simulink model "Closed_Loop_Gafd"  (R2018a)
settings: Solver=ode23s  StartTime=0.0  StopTime=50  RelTol=1e-3  EnableMultiTasking=on
InitFcn:
  | init
StopFcn:
  | pl
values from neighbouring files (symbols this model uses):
  Cyb = -0.0245    [init.m]    (also in lqr_des.m)
  Cydel = [-0.24668,0.24668, 0.47413,-0.47413,0]/100    [init.m]    (also in lqr_des.m = [-0.24668,0.24668, 0.47413,-0.47413]/100)
  Cza = -0.073    [init.m]
  Czdel = [0.51664,0.51664,0.60478,0.60478,0.06]/100    [init.m]
  d2r = pi/180    (= 0.0174532925199)    [init.m]
  Mass = 198.32    [init.m]    (also in lqr_des.m)
  Qbar = 150    [init.m]    (also in lqr_des.m)
  r2d = 180/pi    (= 57.2957795131)    [init.m]    (also in pl.m)
  Sref = 79.069    [init.m]    (also in lqr_des.m)
  V0 = 822.8    [init.m]
undefined symbols (not defined in the file or in its folder): Abfp, Afla, Ardr, Avf, Bbfp, Bfla, Brdr, Bvf, Cbfp, Cfla, Crdr, Cvf, Dbfp, Dfla, Drdr, Dvf, K4axmix, Kpr, Kq

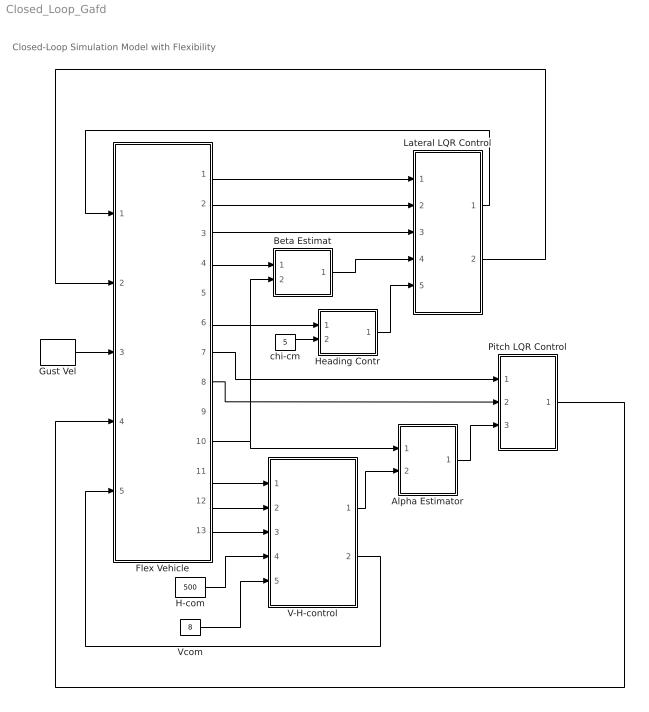
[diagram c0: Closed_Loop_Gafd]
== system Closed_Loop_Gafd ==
  note: Closed-Loop Simulation Model with Flexibility
  Alpha Estimator : Subsystem
  Beta Estimat : Subsystem
  Flex Vehicle : Subsystem
  Gust Vel : DiscretePulseGenerator  PulseType=Time based  Amplitude=160  Period=200  PulseWidth=0.05  PhaseDelay=8
  H-com : Constant  Value=500
  Heading Contr : Subsystem
  Lateral LQR Control : Subsystem
  Pitch LQR Control : Subsystem
  V-H-control : Subsystem
  Vcom : Constant  Value=8
  chi-cm : Constant  Value=5
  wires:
  chi-cm/1 -> Heading Contr/2(chi-cmd)
  Flex Vehicle/2(p) -> Lateral LQR Control/2(p)
  Flex Vehicle/3(r) -> Lateral LQR Control/3(r)
  Flex Vehicle/1(phi) -> Lateral LQR Control/1(phi)
  Flex Vehicle/4(Ny) -> Beta Estimat/1(Ydd)
  Flex Vehicle/6("chi ") -> Heading Contr/1(chi)
  Flex Vehicle/12(Nz) -> V-H-control/2(Az)
  Flex Vehicle/13(dH) -> V-H-control/3(dH)
  Flex Vehicle/11(V-dot) -> V-H-control/1(Vdot)
  Flex Vehicle/10(delt) -> Beta Estimat/2(delta), Alpha Estimator/1(delta)
  Alpha Estimator/1(alphat) -> Pitch LQR Control/3(alfa)
  V-H-control/1(Zdd-com) -> Alpha Estimator/2(Zdd)
  Pitch LQR Control/1(dQ) -> Flex Vehicle/4(dQ)
  Beta Estimat/1(bethat) -> Lateral LQR Control/4(bet)
  Lateral LQR Control/2(dR) -> Flex Vehicle/2(dR)
  Lateral LQR Control/1(dP) -> Flex Vehicle/1(dP)
  V-H-control/2(Throtle) -> Flex Vehicle/5(Ax-cmd)
  Flex Vehicle/8(q) -> Pitch LQR Control/2(q)
  Flex Vehicle/7(thet) -> Pitch LQR Control/1(thet)
  Heading Contr/1(phi-cmd) -> Lateral LQR Control/5(ph-cmd)
  H-com/1 -> V-H-control/4(H-comd)
  Vcom/1 -> V-H-control/5(Vcomd)
  Gust Vel/1 -> Flex Vehicle/3(Gust)

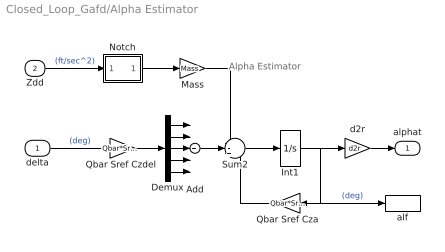
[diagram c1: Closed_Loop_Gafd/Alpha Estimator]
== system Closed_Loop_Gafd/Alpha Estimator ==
  note: Alpha Estimator
  delta : Inport
  Zdd : Inport  Port=2
  Add : Sum  Inputs=+++++
  Demux : Demux  Outputs=5
  Int1 : Integrator
  Mass : Gain  Gain=Mass
  Notch : Subsystem
  Qbar Sref Cza : Gain  Gain=Qbar*Sref*Cza
  "Qbar Sref Czdel " : Gain  Gain=Qbar*Sref*Czdel
  Sum2 : Sum  Inputs=--+
  alf : ToWorkspace  VariableName=alphat  SampleTime=-1
  d2r : Gain  Gain=d2r
  alphat : Outport
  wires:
  Demux/5 -> Add/5
  Demux/4 -> Add/4
  Demux/3 -> Add/3
  Demux/2 -> Add/2
  Demux/1 -> Add/1
  "Qbar Sref Czdel "/1 -> Demux/1
  delta/1 -> "Qbar Sref Czdel "/1  "(deg)"
  Sum2/1 -> Int1/1
  Int1/1 -> d2r/1, alf/1, Qbar Sref Cza/1  "(deg)"
  Qbar Sref Cza/1 -> Sum2/3
  Mass/1 -> Sum2/1
  d2r/1 -> alphat/1
  Add/1 -> Sum2/2
  Zdd/1 -> Notch/1(in)  "(ft/sec^2)"
  Notch/1(ou) -> Mass/1

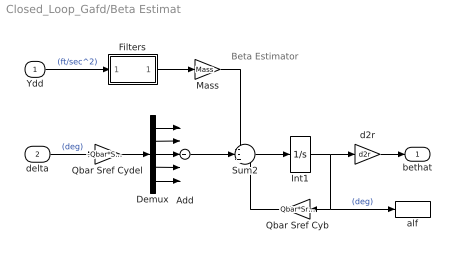
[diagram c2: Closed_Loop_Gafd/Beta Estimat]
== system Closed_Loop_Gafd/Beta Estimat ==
  note: Beta Estimator
  Ydd : Inport
  delta : Inport  Port=2
  Add : Sum  Inputs=+++++
  Demux : Demux  Outputs=5
  Filters : Subsystem
  Int1 : Integrator
  Mass : Gain  Gain=Mass
  Qbar Sref Cyb : Gain  Gain=Qbar*Sref*Cyb
  Qbar Sref Cydel : Gain  Gain=-Qbar*Sref*Cydel
  Sum2 : Sum  Inputs=--+
  alf : ToWorkspace  VariableName=bethat  SampleTime=-1
  d2r : Gain  Gain=d2r
  bethat : Outport
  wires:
  Add/1 -> Sum2/2
  d2r/1 -> bethat/1
  Mass/1 -> Sum2/1
  Ydd/1 -> Filters/1(In)  "(ft/sec^2)"
  Qbar Sref Cyb/1 -> Sum2/3
  Int1/1 -> d2r/1, alf/1, Qbar Sref Cyb/1  "(deg)"
  Sum2/1 -> Int1/1
  delta/1 -> Qbar Sref Cydel/1  "(deg)"
  Qbar Sref Cydel/1 -> Demux/1
  Demux/1 -> Add/1
  Demux/2 -> Add/2
  Demux/3 -> Add/3
  Demux/4 -> Add/4
  Demux/5 -> Add/5
  Filters/1(Ou) -> Mass/1

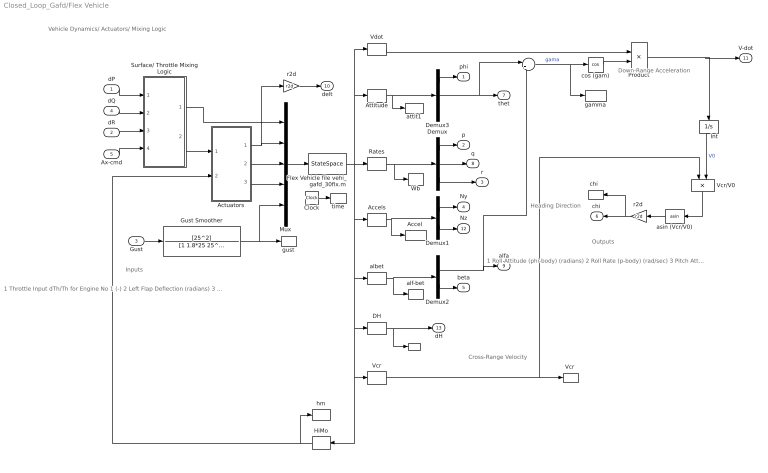
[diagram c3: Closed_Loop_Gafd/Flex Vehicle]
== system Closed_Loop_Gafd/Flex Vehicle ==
  note: 1 Roll Attitude (phi-body) (radians) 2 Roll Rate (p-body) (rad/sec) 3 Pitch Attitude (thet-bdy) (radians) 4 Pitch Rate (q-body) (rad/sec) 5 Yaw Attitude (psi-body) (radians) 6 Yaw Rate (r-body) (rad/sec) 7 Angle of attack, alfa, (radians) 8 Angle of sideslip, beta, (radian) 9 Change in Altitude, delta-h, (feet) 10 Forward Acceleration (V-dot) (ft/sec) 11 Cross Range Velocity (Vcr) (ft/sec) 12 Rate-Gyro # 1, Roll Rate (Body) (rad/sec) 13 Rate-Gyro # 2, Pitch Rate (Body) (rad/sec) 14 Rate-Gyro # 3, Yaw Rate (Body) (rad/sec) 15 Accelerom # 1, (along Y), (ft/sec^2) Translat. Acceler 16 Accelerom # 2, (along Z), (ft/sec^2) Translat. Acceler 17 Hinge Moment for Aero Surface # 1, (ft-lb) 18 Hinge Moment for Aero Surface # 2, (ft-lb) 19 Hinge Moment for Aero Surface # 3, (ft-lb) 20 Hinge Moment for Aero Surface # 4, (ft-lb) 21 Hinge Moment for Aero Surface # 5, (ft-lb)
  note: 1 Throttle Input dTh/Th for Engine No 1 (-) 2 Left Flap Deflection (radians) 3 Right Flap Deflection (radians) 4 Left Rudder Deflection (radians) 5 Right Rudder Deflection (radians) 6 Body Flap Deflection (radians) 7 Left Flap Velocity (rad/sec) 8 Right Flap Velocity (rad/sec) 9 Left Rudder Velocity (rad/sec) 10 Right Rudder Velocity (rad/sec) 11 Body Flap Velocity (rad/sec) 12 Left Flap Acceleration (rad/s^2) 13 Right Flap Acceleration (rad/s^2) 14 Left Rudder Acceleration (rad/s^2) 15 Right Rudder Acceleration (rad/s^2) 16 Body Flap Acceleration (rad/s^2) 17 Wind Gust Azim, Elev Angles=(45.0 90.0) (deg)
  note: Inputs
  note: Outputs
  note: Down-Range Acceleration
  note: Heading Direction
  note: Cross-Range Velocity
  note: Vehicle Dynamics/ Actuators/ Mixing Logic
  dP : Inport
  dR : Inport  Port=2
  Gust : Inport  Port=3
  dQ : Inport  Port=4
  Ax-cmd : Inport  Port=5
  " " : ToWorkspace  VariableName=dH  SampleTime=-1
  "    " : Sum  Inputs=|+-
  "Accel " : ToWorkspace  VariableName=Accel  SampleTime=-1
  Accels : Selector  InputPortWidth=21  IndexOptions=Index vector (dialog)  Indices=[15,16]  OutputSizes=1
  Actuators : Subsystem
  Attitude : Selector  InputPortWidth=21  IndexOptions=Index vector (dialog)  Indices=[1,3,5]  OutputSizes=1
  Clock : Clock
  DH : Selector  InputPortWidth=21  IndexOptions=Index vector (dialog)  Indices=[9]  OutputSizes=1
  Demux : Demux  Outputs=3
  Demux1 : Demux  Outputs=2
  Demux2 : Demux  Outputs=2
  Demux3 : Demux  Outputs=3
  Flex Vehicle file vehi_gafd_30flx.m : StateSpace  A=Avf  B=Bvf  C=Cvf  D=Dvf  InitialCondition=0
  Gust Smoother : TransferFcn  Numerator=[25^2]  Denominator=[1 1.8*25 25^2]
  HiMo : Selector  InputPortWidth=21  IndexOptions=Index vector (dialog)  Indices=[17:21]  OutputSizes=1
  Int : Integrator  InitialCondition=V0
  Mux : Mux  Inputs=[1, 5,5,5, 1]
  Product : Product
  Rates : Selector  InputPortWidth=21  IndexOptions=Index vector (dialog)  Indices=[12:14]  OutputSizes=1
  Surface/ Throttle Mixing Logic : Subsystem
  Vcr : Selector  InputPortWidth=21  IndexOptions=Index vector (dialog)  Indices=[11]  OutputSizes=1
  "Vcr " : ToWorkspace  VariableName=Vcr  SampleTime=-1
  Vcr/V0 : Product  Inputs=*/
  Vdot : Selector  InputPortWidth=21  IndexOptions=Index vector (dialog)  Indices=[10]  OutputSizes=1
  Wb : ToWorkspace  VariableName=Wb  SampleTime=-1
  albet : Selector  InputPortWidth=21  IndexOptions=Index vector (dialog)  Indices=[7,8]  OutputSizes=1
  alf-bet : ToWorkspace  VariableName=albe  SampleTime=-1
  asin (Vcr/V0) : Trigonometry  Operator=asin
  attit1 : ToWorkspace  VariableName=attit  SampleTime=-1
  "chi  " : ToWorkspace  VariableName=chi  SampleTime=-1
  cos (gam) : Trigonometry  Operator=cos
  gamma : ToWorkspace  VariableName=gama  SampleTime=-1
  gust : ToWorkspace  VariableName=gust  SampleTime=-1
  hm : ToWorkspace  VariableName=HM  SampleTime=-1
  r2d : Gain  Gain=r2d
  "r2d " : Gain  Gain=r2d
  time : ToWorkspace  VariableName=time  SampleTime=-1
  phi : Outport
  p : Outport  Port=2
  r : Outport  Port=3
  Ny : Outport  Port=4
  beta : Outport  Port=5
  "chi " : Outport  Port=6
  thet : Outport  Port=7
  q : Outport  Port=8
  alfa : Outport  Port=9
  delt : Outport  Port=10
  V-dot : Outport  Port=11
  Nz : Outport  Port=12
  dH : Outport  Port=13
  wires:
  Mux/1 -> Flex Vehicle file vehi_gafd_30flx.m/1
  Surface/ Throttle Mixing Logic/1(Thro) -> Mux/1
  dP/1 -> Surface/ Throttle Mixing Logic/1(roll)
  dQ/1 -> Surface/ Throttle Mixing Logic/2(ptch)
  dR/1 -> Surface/ Throttle Mixing Logic/3(yaw)
  Ax-cmd/1 -> Surface/ Throttle Mixing Logic/4(Ax)
  r2d/1 -> delt/1
  "r2d "/1 -> "chi "/1, "chi  "/1
  Vcr/V0/1 -> asin (Vcr/V0)/1
  asin (Vcr/V0)/1 -> "r2d "/1
  Product/1 -> V-dot/1, Int/1
  Int/1 -> Vcr/V0/2  "V0"
  "    "/1 -> cos (gam)/1, gamma/1  "gama"
  Surface/ Throttle Mixing Logic/2(delta) -> Actuators/1(del-cmd)
  Actuators/1(delta) -> Mux/2, r2d/1
  Actuators/3(del-ddot) -> Mux/4
  Actuators/2(del-dot) -> Mux/3
  Gust/1 -> Gust Smoother/1
  Clock/1 -> time/1
  Gust Smoother/1 -> gust/1, Mux/5
  Rates/1 -> Wb/1, Demux/1
  Flex Vehicle file vehi_gafd_30flx.m/1 -> Vcr/1, HiMo/1, DH/1, albet/1, Accels/1, Vdot/1, Attitude/1, Rates/1
  HiMo/1 -> hm/1, Actuators/2(HM)
  Demux/1 -> p/1
  Demux/2 -> q/1
  Demux/3 -> r/1
  Accels/1 -> "Accel "/1, Demux1/1
  Demux1/1 -> Ny/1
  Demux1/2 -> Nz/1
  albet/1 -> alf-bet/1, Demux2/1
  Demux2/1 -> "    "/2, alfa/1
  Demux2/2 -> beta/1
  Attitude/1 -> attit1/1, Demux3/1
  Demux3/2 -> "    "/1, thet/1
  Demux3/1 -> phi/1
  DH/1 -> " "/1, dH/1
  cos (gam)/1 -> Product/2
  Vdot/1 -> Product/1
  Vcr/1 -> "Vcr "/1, Vcr/V0/1

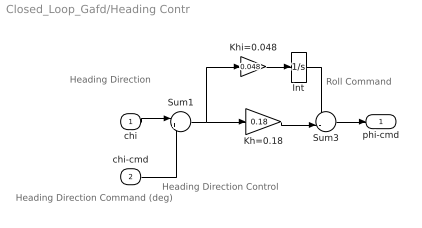
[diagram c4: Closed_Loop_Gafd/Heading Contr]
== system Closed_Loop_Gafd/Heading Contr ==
  note: Heading Direction Control
  note: Heading Direction
  note: Roll Command
  note: Heading Direction Command (deg)
  chi : Inport
  chi-cmd : Inport  Port=2
  Int : Integrator
  Kh=0.18 : Gain  Gain=0.18
  Khi=0.048 : Gain  Gain=0.048
  Sum1 : Sum  Inputs=|+-
  Sum3 : Sum  Inputs=--|
  phi-cmd : Outport
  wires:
  Khi=0.048/1 -> Int/1
  Kh=0.18/1 -> Sum3/2
  Int/1 -> Sum3/1
  Sum3/1 -> phi-cmd/1
  Sum1/1 -> Kh=0.18/1, Khi=0.048/1
  chi/1 -> Sum1/1
  chi-cmd/1 -> Sum1/2

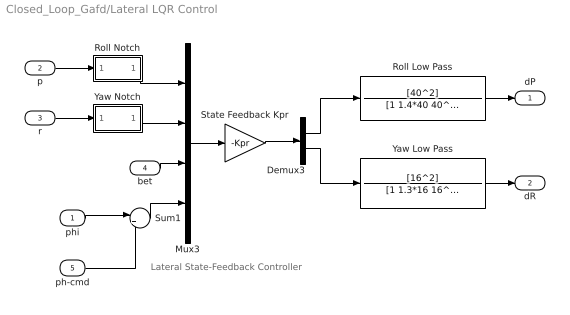
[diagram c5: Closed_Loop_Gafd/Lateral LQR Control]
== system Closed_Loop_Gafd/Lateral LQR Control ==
  note: Lateral State-Feedback Controller
  phi : Inport
  p : Inport  Port=2
  r : Inport  Port=3
  bet : Inport  Port=4
  ph-cmd : Inport  Port=5
  Demux3 : Demux  Outputs=2
  Mux3 : Mux
  Roll Low Pass : TransferFcn  Numerator=[40^2]  Denominator=[1 1.4*40 40^2]
  Roll Notch : Subsystem
  State Feedback Kpr : Gain  Gain=-Kpr  Multiplication=Matrix(K*u) (u vector)
  Sum1 : Sum  Inputs=|+-
  Yaw Low Pass : TransferFcn  Numerator=[16^2]  Denominator=[1 1.3*16 16^2]
  Yaw Notch : Subsystem
  dP : Outport
  dR : Outport  Port=2
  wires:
  Yaw Notch/1(Ot) -> Mux3/2
  Yaw Low Pass/1 -> dR/1
  State Feedback Kpr/1 -> Demux3/1
  Mux3/1 -> State Feedback Kpr/1
  p/1 -> Roll Notch/1(in)
  bet/1 -> Mux3/3
  Demux3/1 -> Roll Low Pass/1
  Sum1/1 -> Mux3/4
  phi/1 -> Sum1/1
  ph-cmd/1 -> Sum1/2
  Roll Notch/1(ou) -> Mux3/1
  r/1 -> Yaw Notch/1(In)
  Demux3/2 -> Yaw Low Pass/1
  Roll Low Pass/1 -> dP/1

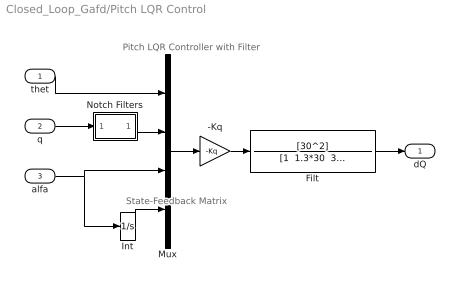
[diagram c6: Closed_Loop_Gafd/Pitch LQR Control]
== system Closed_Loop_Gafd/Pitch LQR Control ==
  note: Pitch LQR Controller with Filter
  note: State-Feedback Matrix
  thet : Inport
  q : Inport  Port=2
  alfa : Inport  Port=3
  -Kq : Gain  Gain=-Kq  Multiplication=Matrix(K*u)
  Filt : TransferFcn  Numerator=[30^2]  Denominator="[1  1.3*30  30^2]"
  Int : Integrator
  Mux : Mux
  Notch Filters : Subsystem
  dQ : Outport
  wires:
  Mux/1 -> -Kq/1
  Int/1 -> Mux/4
  -Kq/1 -> Filt/1
  q/1 -> Notch Filters/1(in)
  thet/1 -> Mux/1
  alfa/1 -> Mux/3, Int/1
  Notch Filters/1(ou) -> Mux/2
  Filt/1 -> dQ/1

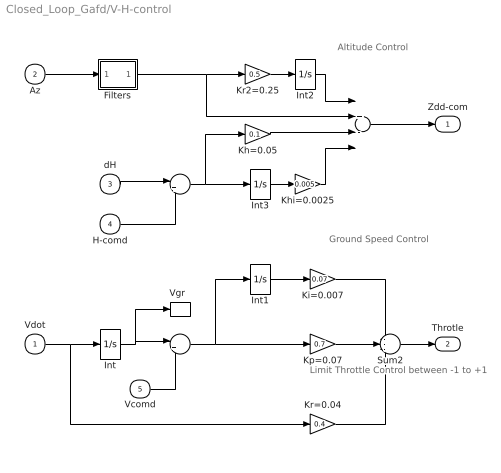
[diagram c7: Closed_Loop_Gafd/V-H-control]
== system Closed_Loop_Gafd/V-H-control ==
  note: Altitude Control
  note: Ground Speed Control
  note: Limit Throttle Control between -1 to +1
  Vdot : Inport
  Az : Inport  Port=2
  dH : Inport  Port=3
  H-comd : Inport  Port=4
  Vcomd : Inport  Port=5
  " " : Sum  Inputs=|+-
  "  " : Sum  Inputs=++--
  "    " : Sum  Inputs=|+-
  Filters : Subsystem
  Int{,1..3} (4 alike) : Integrator
  Kh=0.05 : Gain  Gain=0.1
  Khi=0.0025 : Gain  Gain=0.005
  Ki=0.007 : Gain  Gain=0.07
  Kp=0.07 : Gain  Gain=0.7
  Kr2=0.25 : Gain  Gain=0.5
  Kr=0.04 : Gain  Gain=0.4
  Sum2 : Sum  Inputs=---
  "Vgr  " : ToWorkspace  VariableName=Vgr  SampleTime=-1
  Zdd-com : Outport
  Throtle : Outport  Port=2
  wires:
  Khi=0.0025/1 -> "  "/4
  Int3/1 -> Khi=0.0025/1
  " "/1 -> Kh=0.05/1, Int3/1
  "  "/1 -> Zdd-com/1
  Int2/1 -> "  "/1
  Kr2=0.25/1 -> Int2/1
  Kh=0.05/1 -> "  "/3
  H-comd/1 -> " "/2
  dH/1 -> " "/1
  Vcomd/1 -> "    "/2
  "    "/1 -> Int1/1, Kp=0.07/1
  Int/1 -> "    "/1, "Vgr  "/1
  Int1/1 -> Ki=0.007/1
  Ki=0.007/1 -> Sum2/1
  Kp=0.07/1 -> Sum2/2
  Kr=0.04/1 -> Sum2/3
  Sum2/1 -> Throtle/1
  Vdot/1 -> Kr=0.04/1, Int/1
  Filters/1(ou) -> "  "/2, Kr2=0.25/1
  Az/1 -> Filters/1(in)

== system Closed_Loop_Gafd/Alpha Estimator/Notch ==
  note: Notch Filters
  in : Inport
  Notch 79 rad : TransferFcn  Numerator="[1  0.03*79  79^2]"  Denominator="[1  0.4*79  79^2]"
  ou : Outport
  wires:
  Notch 79 rad/1 -> ou/1
  in/1 -> Notch 79 rad/1

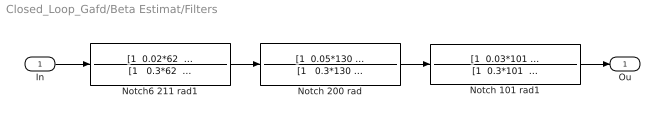
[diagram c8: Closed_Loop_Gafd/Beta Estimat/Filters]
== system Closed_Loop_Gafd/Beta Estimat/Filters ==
  In : Inport
  Notch 101 rad1 : TransferFcn  Numerator="[1  0.03*101  101^2]"  Denominator="[1  0.3*101  101^2]"
  Notch 200 rad : TransferFcn  Numerator="[1  0.05*130  130^2]"  Denominator="[1   0.3*130  130^2]"
  Notch6 211 rad1 : TransferFcn  Numerator="[1  0.02*62  62.7^2]"  Denominator="[1   0.3*62  62.7^2]"
  Ou : Outport
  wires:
  Notch 200 rad/1 -> Notch 101 rad1/1
  Notch 101 rad1/1 -> Ou/1
  Notch6 211 rad1/1 -> Notch 200 rad/1
  In/1 -> Notch6 211 rad1/1

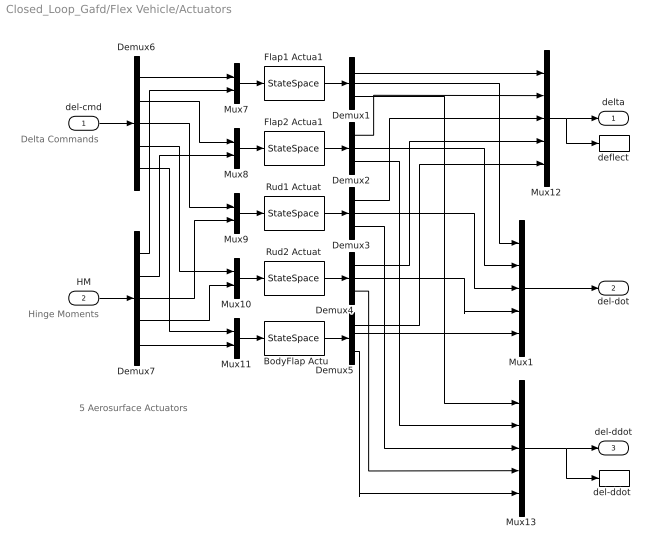
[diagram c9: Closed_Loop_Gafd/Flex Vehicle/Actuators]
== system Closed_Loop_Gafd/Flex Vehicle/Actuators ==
  note: 5 Aerosurface Actuators
  note: Hinge Moments
  note: Delta Commands
  del-cmd : Inport
  HM : Inport  Port=2
  BodyFlap Actu : StateSpace  A=Abfp  B=Bbfp  C=Cbfp  D=Dbfp  InitialCondition=0
  Demux{1..5} (5 alike) : Demux  Outputs=3
  Demux6 : Demux  Outputs=5
  Demux7 : Demux  Outputs=5
  Flap1 Actua1 : StateSpace  A=Afla  B=Bfla  C=Cfla  D=Dfla  InitialCondition=0
  Flap2 Actua1 : StateSpace  A=Afla  B=Bfla  C=Cfla  D=Dfla  InitialCondition=0
  Mux1 : Mux  Inputs=5
  Mux{7..11} (5 alike) : Mux  Inputs=2
  Mux12 : Mux  Inputs=5
  Mux13 : Mux  Inputs=5
  Rud1 Actuat : StateSpace  A=Ardr  B=Brdr  C=Crdr  D=Drdr  InitialCondition=0
  Rud2 Actuat : StateSpace  A=Ardr  B=Brdr  C=Crdr  D=Drdr  InitialCondition=0
  deflect : ToWorkspace  VariableName=delta  SampleTime=-1
  "del-ddot " : ToWorkspace  VariableName=deldd  SampleTime=-1
  delta : Outport
  del-dot : Outport  Port=2
  del-ddot : Outport  Port=3
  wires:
  Mux7/1 -> Flap1 Actua1/1
  Flap1 Actua1/1 -> Demux1/1
  Mux8/1 -> Flap2 Actua1/1
  Flap2 Actua1/1 -> Demux2/1
  Mux9/1 -> Rud1 Actuat/1
  Rud1 Actuat/1 -> Demux3/1
  Mux10/1 -> Rud2 Actuat/1
  Rud2 Actuat/1 -> Demux4/1
  Mux11/1 -> BodyFlap Actu/1
  BodyFlap Actu/1 -> Demux5/1
  Demux6/1 -> Mux7/1
  Demux6/2 -> Mux8/1
  Demux6/3 -> Mux9/1
  Demux6/4 -> Mux10/1
  Demux6/5 -> Mux11/1
  Demux7/5 -> Mux11/2
  Demux7/4 -> Mux10/2
  Demux7/3 -> Mux9/2
  Demux7/2 -> Mux8/2
  Demux7/1 -> Mux7/2
  Demux1/1 -> Mux12/1
  Demux2/1 -> Mux12/2
  Demux3/1 -> Mux12/3
  Demux4/1 -> Mux12/4
  Demux5/1 -> Mux12/5
  Demux4/3 -> Mux13/4
  Demux3/3 -> Mux13/3
  Demux2/3 -> Mux13/2
  Demux1/3 -> Mux13/1
  Demux1/2 -> Mux1/1
  Mux12/1 -> deflect/1, delta/1
  del-cmd/1 -> Demux6/1
  Demux2/2 -> Mux1/2
  Demux3/2 -> Mux1/3
  Demux4/2 -> Mux1/4
  Mux13/1 -> "del-ddot "/1, del-ddot/1
  Demux5/2 -> Mux1/5
  Demux5/3 -> Mux13/5
  Mux1/1 -> del-dot/1
  HM/1 -> Demux7/1

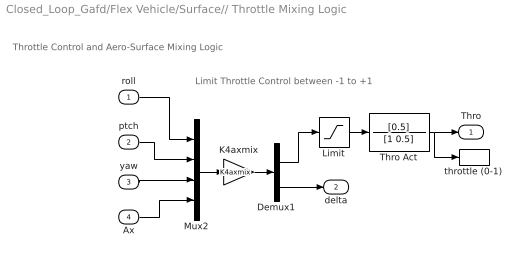
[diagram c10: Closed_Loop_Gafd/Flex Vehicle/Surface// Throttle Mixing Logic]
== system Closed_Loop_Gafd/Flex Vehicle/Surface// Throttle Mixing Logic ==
  note: Limit Throttle Control between -1 to +1
  note: Throttle Control and Aero-Surface Mixing Logic
  roll : Inport
  ptch : Inport  Port=2
  yaw : Inport  Port=3
  Ax : Inport  Port=4
  Demux1 : Demux  Outputs=[1, 5]
  K4axmix : Gain  Gain=K4axmix  Multiplication=Matrix(K*u) (u vector)
  Limit : Saturate  UpperLimit=1  LowerLimit=-1
  Mux2 : Mux
  Thro Act : TransferFcn  Numerator=[0.5]  Denominator=[1 0.5]
  throttle (0-1) : ToWorkspace  VariableName=Thro  SampleTime=-1
  Thro : Outport
  delta : Outport  Port=2
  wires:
  Thro Act/1 -> throttle (0-1)/1, Thro/1
  Limit/1 -> Thro Act/1
  K4axmix/1 -> Demux1/1
  Mux2/1 -> K4axmix/1
  Demux1/1 -> Limit/1
  Demux1/2 -> delta/1
  roll/1 -> Mux2/1
  Ax/1 -> Mux2/4
  yaw/1 -> Mux2/3
  ptch/1 -> Mux2/2

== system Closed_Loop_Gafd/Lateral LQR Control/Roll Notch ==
  in : Inport
  Notch 63 rad1 : TransferFcn  Numerator="[1  0.02*62  62.7^2]"  Denominator="[1   0.3*62  62.7^2]"
  ou : Outport
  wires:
  Notch 63 rad1/1 -> ou/1
  in/1 -> Notch 63 rad1/1

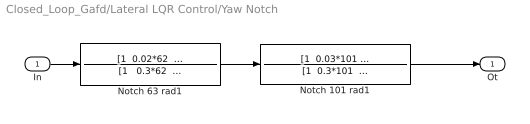
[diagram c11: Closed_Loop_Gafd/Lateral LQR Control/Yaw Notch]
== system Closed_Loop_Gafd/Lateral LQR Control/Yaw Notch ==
  In : Inport
  Notch 101 rad1 : TransferFcn  Numerator="[1  0.03*101  101^2]"  Denominator="[1  0.3*101  101^2]"
  Notch 63 rad1 : TransferFcn  Numerator="[1  0.02*62  62.7^2]"  Denominator="[1   0.3*62  62.7^2]"
  Ot : Outport
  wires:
  Notch 101 rad1/1 -> Ot/1
  Notch 63 rad1/1 -> Notch 101 rad1/1
  In/1 -> Notch 63 rad1/1

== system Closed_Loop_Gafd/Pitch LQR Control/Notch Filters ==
  note: Notch Filters
  in : Inport
  Notch 106 rad : TransferFcn  Numerator="[1  0.02*106  107^2]"  Denominator="[1  0.4*106  107^2]"
  Notch 79 rad : TransferFcn  Numerator="[1  0.02*79  78.5^2]"  Denominator="[1  0.4*79  78.5^2]"
  ou : Outport
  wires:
  Notch 79 rad/1 -> Notch 106 rad/1
  Notch 106 rad/1 -> ou/1
  in/1 -> Notch 79 rad/1

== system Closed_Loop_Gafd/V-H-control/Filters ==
  in : Inport
  Notch 106 rad : TransferFcn  Numerator="[1  0.02*106  107^2]"  Denominator="[1  0.4*106  107^2]"
  ou : Outport
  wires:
  Notch 106 rad/1 -> ou/1
  in/1 -> Notch 106 rad/1
